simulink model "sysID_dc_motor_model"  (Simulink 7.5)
settings: Solver=ode45  StartTime=0.0  StopTime=100  RelTol=1e-3
libraries: simulink x1

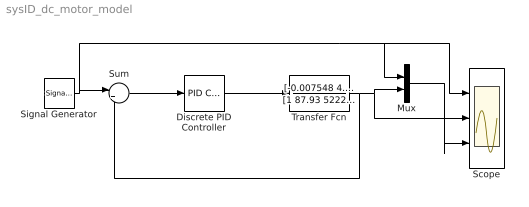
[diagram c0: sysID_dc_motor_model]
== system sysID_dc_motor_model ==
  Discrete PID Controller : simulink/Continuous/PID Controller  DialogController=pidpack.PIDConfig.pidDDGCreate  DialogControllerArgs=DataTag0  SystemSampleTime=-1  Controller=PID  TimeDomain=Continuous-time  SampleTime=1  IntegratorMethod=Forward Euler  FilterMethod=Forward Euler  Form=Parallel  P=0  I=5.44113062499075  D=0  N=100  InitialConditionSource=internal  InitialConditionForIntegrator=0  InitialConditionForFilter=0  ExternalReset=none  LimitOutput=off  UpperSaturationLimit=inf  LowerSaturationLimit=-inf  LinearizeAsGain=off  AntiWindupMode=none  Kb=1  TrackingMode=off  Kt=1  PParamMin=[]  PParamMax=[]  IParamMin=[]  IParamMax=[]  DParamMin=[]  DParamMax=[]  NParamMin=[]  NParamMax=[]  KbParamMin=[]  KbParamMax=[]  KtParamMin=[]  KtParamMax=[]  POutMin=[]  POutMax=[]  IOutMin=[]  IOutMax=[]  DOutMin=[]  DOutMax=[]  NOutMin=[]  NOutMax=[]  KbOutMin=[]  KbOutMax=[]  KtOutMin=[]  KtOutMax=[]  IntegratorOutMin=[]  IntegratorOutMax=[]  FilterOutMin=[]  FilterOutMax=[]  SumOutMin=[]  SumOutMax=[]  SumI1OutMin=[]  SumI1OutMax=[]  SumI2OutMin=[]  SumI2OutMax=[]  SumI3OutMin=[]  SumI3OutMax=[]  SumDOutMin=[]  SumDOutMax=[]  SaturationOutMin=[]  SaturationOutMax=[]  IntegratorContinuousStateAttributes=''  IntegratorStateMustResolveToSignalObject=off  IntegratorRTWStateStorageClass=Auto  FilterContinuousStateAttributes=''  FilterStateMustResolveToSignalObject=off  FilterRTWStateStorageClass=Auto
  Mux : Mux  Inputs=2
  Scope : Scope  NumInputPorts=3
  Signal Generator : SignalGenerator  WaveForm=square  Amplitude=4000  Frequency=0.1
  Sum : Sum  Inputs=|+-  OutDataType=fixdt(1, 16)  OutScaling=2^0
  Transfer Fcn : TransferFcn  Numerator=[-0.007548 4.41 -871.1 5.767e4]  Denominator=[1 87.93 5222 9.627e4]
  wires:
  Signal Generator/1 -> Sum/1, Mux/1, Scope/1
  Sum/1 -> Discrete PID Controller/1
  Discrete PID Controller/1 -> Transfer Fcn/1
  Transfer Fcn/1 -> Sum/2, Mux/2, Scope/2
  Mux/1 -> Scope/3
